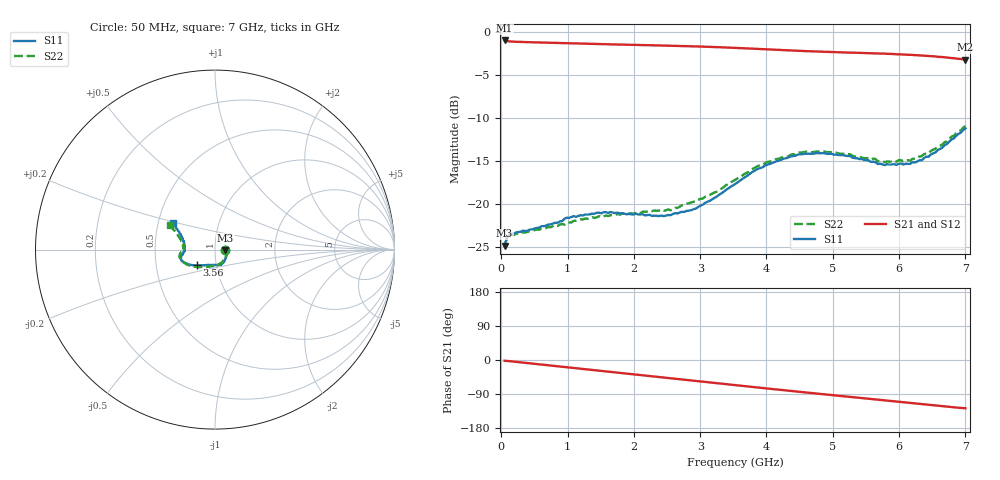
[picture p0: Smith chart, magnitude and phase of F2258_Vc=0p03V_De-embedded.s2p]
! Integrated Device Technology
! Corporate Headquarters
! 6024 Silver Creek Valley Road
! San Jose, CA 95138  USA
! Phone:  1-408-284-8200
! Toll Free:  1-800-223-1366
! Webpage:  http://www.idt.com/
! Timing and RF Division
! 515 Groton Road, Suite 102
! Westford, MA 01886-6024
! Device:  F2258
! Description: Voltage Variable RF Attenuator
! Frequency:  50.0 -  6000.00 MHz
! Package:  3x3 mm Thin QFN Plastic Package: 16 pin
! Ports:  2 RF, 2 DC
!  Pin  1  = NC
!  Pin  2  = NC
!  Pin  3  = RF2  = Port 2
!  Pin  4  = GND
!  Pin  5  = Vdd
!  Pin  6  = NC
!  Pin  7  = VCTRL
!  Pin  8  = NC
!  Pin  9  = GND
!  Pin 10  = RF1  = Port 1
!  Pin 11  = NC
!  Pin 12  = NC
!  Pin 13  = NC
!  Pin 14  = NC
!  Pin 15  = NC
!  Pin 16  = NC
! Vcntrl:  0.030 Volts
! Vdd:  +3.300 Volts
! Current:  1.076 mA
! Data:  The device was measured on a the F2258 evaluation board which has
!  individual transmission lines to the RF pins.  Data was collected
!  using a calibrated network analyzer.  The evaluation board was
!  de-embedded using a TRL calibration technique.
!  The reference plane is the edge of the package pin.
! Misc:  SN 10
!  Action Tracker AT0285
! Date Measured:  2014-12-10
! Date:  2016-01-13  MJV
! Note:
!  Integrated Device Technology supplies this data as a sample of measured
!  data at the package pin for this product.  Your particular data for this
!  product may vary.
!  Data was taken at 25 degrees C.
!  Integrated Device Technology reserves the right to change this data at anytime.
!Freq_(GHz)  S11M_(dB)  S11P_(deg)  S21M_(dB)  S21P_(deg)  S12M_(dB)  S12P_(deg)  S22M_(dB)  S22P_(deg)
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# GHz S dB R 50
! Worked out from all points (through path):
!   201 points, 50 MHz to 7 GHz, reference 50 ohm
!   highest |S21| = -0.96 dB at 50 MHz (marker M1); lowest = -3.2 dB at 7 GHz (marker M2)
!   group delay of S21, straight-line fit = 50.5 ps
!   lowest |S11| = -24.9 dB at 50 MHz (marker M3), VSWR 1.12, Z = 56 - j0.39 ohm
!   |S11| at or under -10 dB: start of sweep to end of sweep
!   |S22| runs from -24.9 to -10.9 dB; largest |S21 - S12| = 0.00042
!   S11 on the Smith chart (normalised r, x): 50 MHz: 1.12, -0.01; 3.56 GHz: 0.81, -0.14; 7 GHz: 0.60, +0.19
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0.05  -24.87 -3.5  -0.96 -1.9  -0.96 -1.9  -24.92 -3.1
0.08475  -23.90 -6.0  -1.03 -2.4  -1.03 -2.4  -23.98 -5.5
0.15425  -23.42 -9.3  -1.08 -3.6  -1.08 -3.6  -23.60 -9.4
0.71025  -22.39 -37.2  -1.22 -14.1  -1.22 -14.1  -22.69 -38.6
0.98825  -21.61 -51.0  -1.27 -19.3  -1.27 -19.3  -22.18 -54.7
1.2315  -21.35 -59.3  -1.32 -23.8  -1.32 -23.8  -21.80 -63.7
1.6485  -20.95 -71.0  -1.41 -31.4  -1.41 -31.4  -21.31 -76.7
2.37825  -21.42 -92.5  -1.54 -44.7  -1.54 -44.7  -20.78 -94.3
2.552  -21.32 -98.5  -1.57 -48.0  -1.57 -48.0  -20.74 -99.6
2.93425  -20.53 -115.1  -1.65 -55.1  -1.65 -55.1  -19.73 -112.9
3.525  -17.69 -137.8  -1.82 -66.2  -1.82 -66.2  -17.21 -135.6
3.55975  -17.50 -138.8  -1.83 -66.9  -1.83 -66.9  -17.03 -136.5
4.0115  -15.43 -151.4  -2.00 -75.2  -2.00 -75.2  -15.12 -151.0
4.46325  -14.28 -159.8  -2.16 -83.4  -2.16 -83.4  -14.07 -162.0
4.7065  -14.15 -163.0  -2.23 -87.7  -2.23 -87.6  -13.96 -166.3
5.2625  -14.43 -170.0  -2.38 -97.4  -2.38 -97.3  -14.21 -174.3
5.6795  -15.35 -176.8  -2.47 -104.6  -2.47 -104.6  -15.03 -179.6
5.85325  -15.42 179.0  -2.52 -107.8  -2.52 -107.8  -15.06 175.7
6.166  -15.34 171.2  -2.63 -113.4  -2.63 -113.3  -14.97 169.8
6.33975  -14.93 164.9  -2.71 -116.5  -2.71 -116.5  -14.43 165.5
6.722  -13.01 153.3  -2.94 -123.1  -2.94 -123.1  -12.71 156.4
7  -11.20 147.9  -3.19 -127.4  -3.19 -127.4  -10.92 151.5
